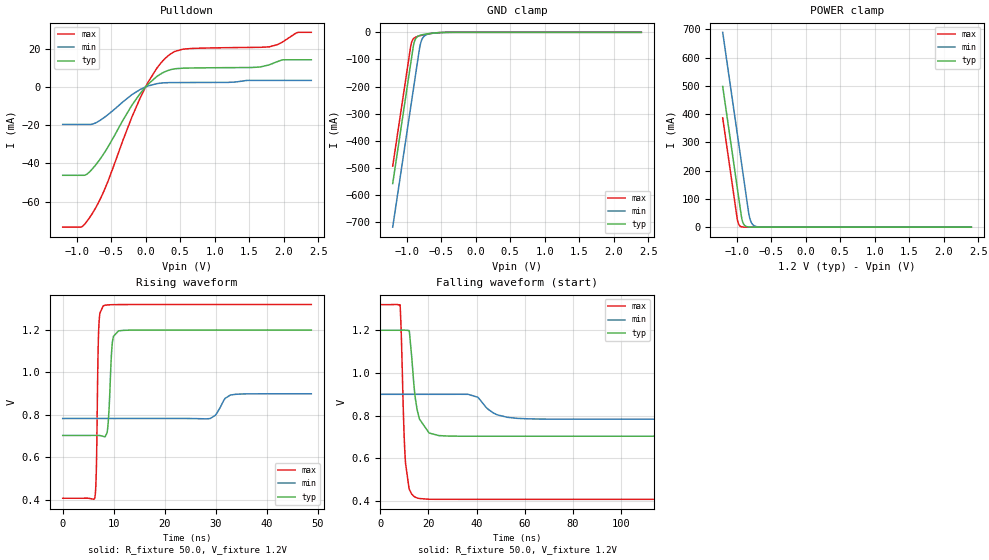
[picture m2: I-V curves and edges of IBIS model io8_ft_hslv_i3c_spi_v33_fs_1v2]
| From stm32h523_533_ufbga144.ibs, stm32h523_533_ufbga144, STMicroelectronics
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[Model]   io8_ft_hslv_i3c_spi_v33_fs_1v2
Model_type I/O_open_drain
Polarity   Non-Inverting
Enable   Active-Low
| CAP_THRESHOLD on pad IOFT is "UDTCAPC" :
| Rising=20.0% of vddiom   Falling=80.0% of vddiom
| C_comp min and max val. don't necessarily correlate with the min and max pvt
| but are the smallest and greatest pad capacitance found.
| var   typ   min   max
C_comp   3.39575pF  3.37230pF  3.42685pF
|C_comp_pulldown   3.39575pF  3.37230pF  3.42685pF
Vinl = 450.0mV
Vinh = 660.0mV
Vmeas = 600.0mV   | Reference voltage for timing measurements
Cref  = 50.0pF   | Timing specification test load capacitance value
Rref  = 1.0MOhm   | Timing specification test load resistance value
Vref  = 660.0mV   | Timing specification test load voltage
[Model Spec]
| TIME_THRESHOLD on pin ZII2CV11 is "CMOS" :
| Rising=40.0% of vdd   Falling=60.0% of vdd
Vinl 437.80000mV 335.80000mV 479.80000mV
Vinh 728.20000mV 529.20000mV 807.20000mV
| variable   typ   min   max
[Temperature Range] 25.0 125.0 -40.0
| variable   typ   min   max
[Voltage Range] 1.2V 900.0mV 1.32V
| variable   typ   min   max
[POWER Clamp Reference] 1.2V 900.0mV 1.32V
| variable   typ   min   max
[GND Clamp Reference] 0V 0V 0V
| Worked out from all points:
|   slope of the pulldown table from 0 to 0.18 V, typ, clamps not added: 30.6 ohm
|   GND clamp passes 1 mA (typ) near -0.52 V on its own axis
|   POWER clamp passes 1 mA (typ) near -0.84 V on its own axis
|   rising waveform, R_fixture 50.0, V_fixture 1.2V: 20-80 % time 575ps typ, 1.64ns min, 337ps max; typ from 0.704 V to 1.2 V
|   falling waveform, R_fixture 50.0, V_fixture 1.2V: 20-80 % time 2.99ns typ, 6.82ns min, 1.58ns max; typ from 1.2 V to 0.704 V
[POWER Clamp]
-1.2V     497.8mA    689.2mA    386.5mA
-990mV    140.8mA    332.2mA    29.53mA
-980mV    123.8mA    315.2mA    17.95mA
-960mV    89.81mA    281.2mA    6.634mA
-930mV    38.81mA    230.2mA    1.49mA
-900mV    12.07mA    179.2mA    334.8uA
-870mV    3.756mA    128.2mA    75.22uA
-820mV    536.4uA    44.98mA    6.246uA
-790mV    166.9uA    18.76mA    1.403uA
-750mV    35.18uA    5.846mA    191.8nA
-590mV    70.08nA    55uA       163.4pA
2.4V      0A         0A         0A
[GND Clamp]
-1.2V     -558.2mA   -719mA     -494.1mA
-940mV    -116.2mA   -277mA     -52.06mA
-930mV    -99.19mA   -260mA     -39.94mA
-900mV    -49.1mA    -209mA     -23.76mA
-880mV    -30.14mA   -175mA     -19.6mA
-850mV    -17.82mA   -124mA     -16.09mA
-810mV    -11.73mA   -56.78mA   -12.91mA
-780mV    -9.444mA   -28.21mA   -10.92mA
-740mV    -7.291mA   -13.16mA   -8.574mA
-640mV    -3.573mA   -4.171mA   -3.954mA
-380mV    -61.75uA   -230.3uA   -20.32uA
2.4V      3.863nA    718.6nA    150.6pA
| variable   typ   min   max
[Pullup Reference] 1.2V 900.0mV 1.32V
| variable   typ   min   max
[Pulldown Reference] 0V 0V 0V
[Pulldown]
-1.2V     -46.17mA   -19.62mA   -73.27mA
-930mV    -46.17mA   -19.62mA   -73.18mA
-770mV    -42.8mA    -19.41mA   -66.04mA
-570mV    -32.88mA   -15.18mA   -51.58mA
-80mV     -3.488mA   -1.363mA   -5.887mA
160mV     5.368mA    1.686mA    9.621mA
340mV     8.782mA    2.251mA    16.66mA
540mV     9.805mA    2.305mA    19.74mA
1.79V     11.53mA    3.428mA    20.94mA
1.98V     14.11mA    3.428mA    23.43mA
2.2V      14.2mA     3.428mA    28.44mA
2.4V      14.2mA     3.428mA    28.54mA
[Ramp]
dV/dt_r 297.78741mV/573.11301ps 69.82839mV/1.62322ns 547.12635mV/334.19986ps
dV/dt_f 297.80519mV/2.91364ns 69.92314mV/6.70906ns 547.1393mV/1.5758ns
R_load = 50.0
| Removed startup time: 0s 0s 0s  .
| Removed end time: 48.75ns.
[Rising Waveform]
R_fixture   = 50.0
V_fixture   = 1.2V
V_fixture_min = 900.0mV
V_fixture_max = 1.32V
0s        703.7mV    783.5mV    408.1mV
6.3ns     703.8mV    783.5mV    410.9mV
6.6ns     703.8mV    783.5mV    545.4mV
6.9ns     703.7mV    783.5mV    1.05V
7.05ns    703.6mV    783.5mV    1.198V
7.95ns    699.3mV    783.5mV    1.314V
8.85ns    744.9mV    783.5mV    1.318V
9.8ns     1.152V     783.5mV    1.319V
10.95ns   1.196V     783.5mV    1.32V
48.75ns   1.2V       899.8mV    1.32V
| Removed startup time: 0s 0s 0s  .
| Removed end time: 198.75ns.
[Falling Waveform]
R_fixture   = 50.0
V_fixture   = 1.2V
V_fixture_min = 900.0mV
V_fixture_max = 1.32V
0s        1.2V       900mV      1.32V
8.2ns     1.2V       900mV      1.318V
8.75ns    1.2V       900mV      1.171V
9.8ns     1.2V       900mV      741.9mV
10.5ns    1.2V       900mV      576mV
12.1ns    1.192V     900mV      454.3mV
15.3ns    828.2mV    900mV      414.5mV
24.35ns   706.7mV    900mV      408.1mV
56.8ns    703.7mV    787.4mV    408.1mV
198.8ns   703.7mV    783.5mV    408.1mV
